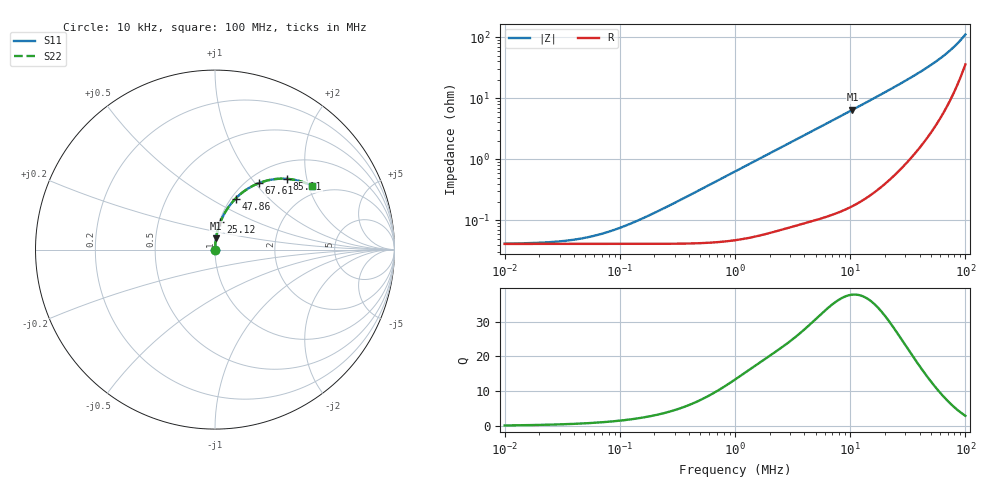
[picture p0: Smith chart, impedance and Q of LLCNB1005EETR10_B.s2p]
! LLCNB1005EETR10_B  S-PARAMETER MODEL  ( Standard Model )
! Model Generated by TAIYO YUDEN Corporation (http://www.ty-top.com)
! Version 1.0
! TAIYO YUDEN Control No. 190130
! Copyright(c) 2019 TAIYO YUDEN CO.,LTD. All Rights Reserved.
! Product Description (link to TY-COMPAS)
! https://ds.yuden.co.jp/TYCOMPAS/or/detail?pn=LLCNB1005EETR10MB&u=M
! Products Name : Inductors
! Characteristics :
!  Inductance : 0.1 [uH] , SRF(min) : - [Hz] , DC Resistance(max) : 50 [mOhm]
!  Rated Current : Saturation  2.0 [A] (dL = 30 [%]), Temp Rise  2.0 [A] (dT = 40 [degC])
!  Case Size : 1.0 x 0.5 / 0.039 x 0.02 [mm/inch] , Thickness : 0.55 / 0.022 [mm/inch]
!  (Conditions: Temperature = 25 [degC] , DC Bias Current = 0 [A])
! External Node Assignments :
!  1  o---GGG---o  2
! GND o---------o GND
! Frequency Range : 10kHz  -  100MHz  [ 402 STEP ]
# MHz S RI R 50
! Freq[MHz].  S11 Real  S11 Imag  S21 Real  S21 Imag  S12 Real  S12 Imag  S22 Real  S22 Imag
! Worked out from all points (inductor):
!   401 points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, 10 kHz to 100 MHz, reference 50 ohm
!   read as one part in series: L = 100 nH near 199.5 kHz
!   highest Q = 37.8 at 10.47 MHz (marker M1), where L = 98 nH
!   S11 on the Smith chart (normalised r, x): 10 kHz: 1.00, +0.00; 25.12 MHz: 1.01, +0.32; 47.86 MHz: 1.05, +0.66; 67.61 MHz: 1.14, +1.05; 85.11 MHz: 1.33, +1.53; 100 MHz: 1.71, +2.09
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0.01  0.00041 6.28e-05  0.9996 -6.28e-05  0.9996 -6.28e-05  0.00041 6.28e-05
0.025119  0.00041 0.000158  0.9996 -0.000158  0.9996 -0.000158  0.00041 0.000158
0.034674  0.00041 0.000218  0.9996 -0.000218  0.9996 -0.000218  0.00041 0.000218
0.046774  0.00041 0.000294  0.9996 -0.000294  0.9996 -0.000294  0.00041 0.000294
0.066069  0.00041 0.000415  0.9996 -0.000415  0.9996 -0.000415  0.00041 0.000415
0.095499  0.00041 0.0006  0.9996 -0.0006  0.9996 -0.0006  0.00041 0.0006
0.138038  0.000411 0.000867  0.9996 -0.000867  0.9996 -0.000867  0.000411 0.000867
0.218776  0.000413 0.00138  0.9996 -0.00138  0.9996 -0.00138  0.000413 0.00138
1  0.00051 0.00628  0.9995 -0.00628  0.9995 -0.00628  0.00051 0.00628
4.677351  0.0018 0.0288  0.9982 -0.0288  0.9982 -0.0288  0.0018 0.0288
10.47128  0.00583 0.064  0.9942 -0.064  0.9942 -0.064  0.00583 0.064
15.48817  0.0117 0.0945  0.9883 -0.0945  0.9883 -0.0945  0.0117 0.0945
21.87762  0.0227 0.1333  0.9773 -0.1333  0.9773 -0.1333  0.0227 0.1333
25.11886  0.0299 0.1528  0.9701 -0.1528  0.9701 -0.1528  0.0299 0.1528
36.30781  0.0635 0.2193  0.9365 -0.2193  0.9365 -0.2193  0.0635 0.2193
47.86301  0.1146 0.2841  0.8854 -0.2841  0.8854 -0.2841  0.1146 0.2841
57.54399  0.1717 0.332  0.8283 -0.332  0.8283 -0.332  0.1717 0.332
67.6083  0.2455 0.3708  0.7545 -0.3708  0.7545 -0.3708  0.2455 0.3708
75.85776  0.3155 0.3901  0.6845 -0.3901  0.6845 -0.3901  0.3155 0.3901
85.1138  0.4009 0.3943  0.5991 -0.3943  0.5991 -0.3943  0.4009 0.3943
95.49926  0.498 0.3736  0.502 -0.3736  0.502 -0.3736  0.498 0.3736
100  0.538 0.3563  0.462 -0.3563  0.462 -0.3563  0.538 0.3563
